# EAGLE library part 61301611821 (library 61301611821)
WURTH ELEKTRONIK - 61301611821 - PCB Receptacle, Board-to-Board, 2.54 mm, 1 Rows, 16 Contacts, Through Hole Mount, WR-PHD Series Source: Datasheet
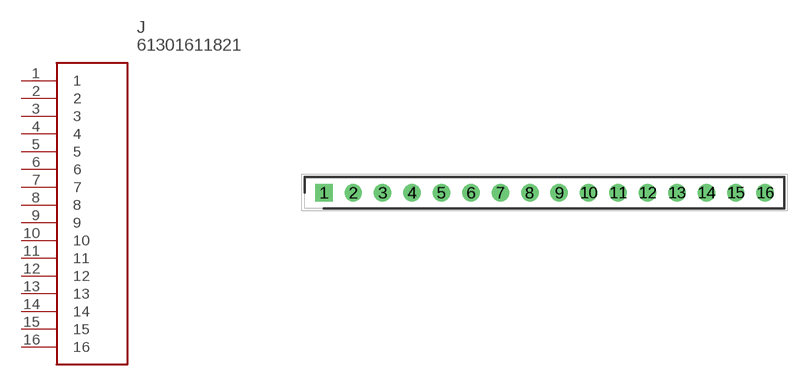
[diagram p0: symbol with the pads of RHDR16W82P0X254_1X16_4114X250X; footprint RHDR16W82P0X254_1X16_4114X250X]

Designator prefix J

## 61301611821 (Description: WURTH ELEKTRONIK - 61301611821 - PCB Receptacle, Board-to-Board, 2.54 mm, 1 Rows, 16 Contacts, Through Hole Mount, WR-PHD Series; Height: 8.65mm; Manufacturer_Name: Wurth Elektronik; Manufacturer_Part_Number: 61301611821; Mouser_Part_Number: 710-61301611821; Mouser_Price-Stock: https://www.mouser.co.uk/ProductDetail/Wurth-Elektronik/61301611821?qs=xZ%2FP%252Ba9zWqYIxo6RU%252B1Wuw%3D%3D)  [RHDR16W82P0X254_1X16_4114X250X]
1  1
2  2
3  3
4  4
5  5
6  6
7  7
8  8
9  9
10  10
11  11
12  12
13  13
14  14
15  15
16  16

## Footprint RHDR16W82P0X254_1X16_4114X250X (pad centres in mm)
61301611821
drill 1 pad 1.5 square: 1 0,0
drill 1 pad 1.5: 2 2.54,0; 3 5.08,0; 4 7.62,0; 5 10.16,0; 6 12.7,0; 7 15.24,0; 8 17.78,0; 9 20.32,0; 10 22.86,0; 11 25.4,0; 12 27.94,0; 13 30.48,0; 14 33.02,0; 15 35.56,0; 16 38.1,0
